PROGRAM MAIN
VAR
	
	fbProxyPLCCalculationTcComModule: FB_ProxyPLCCalculationTcComModule;
	
	i 		: INT;	
	a 		: INT := 10;
	b 		: INT := 7;
	nSum 	: INT; // a + b
	nDiff 	: INT; // a - b

	hrCalc 	: HRESULT;

	bInit	: BOOL;
	hr		:HRESULT;
END_VAR

i := i + 1;

IF bInit THEN
	fbProxyPLCCalculationTcComModule.AfterProviderInit(TC_GLOBAL_IID_LIST.IID_I_Calculation);
	bInit:= FALSE;
END_IF

IF fbProxyPLCCalculationTcComModule.ip <> 0 THEN
	fbProxyPLCCalculationTcComModule.Cyclic();
	hrCalc := fbProxyPLCCalculationTcComModule.ip.Addition(a,b,nSum);
	hrCalc := fbProxyPLCCalculationTcComModule.ip.Subtraction(a,b,nDiff);
END_IF

END_PROGRAM
